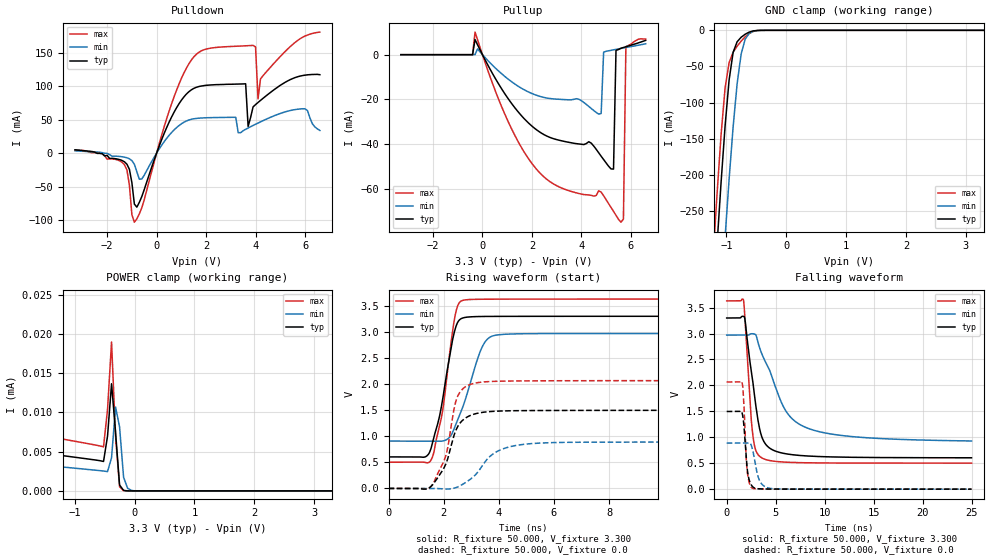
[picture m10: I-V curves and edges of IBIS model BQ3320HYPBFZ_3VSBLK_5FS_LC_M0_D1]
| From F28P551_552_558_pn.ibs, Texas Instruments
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|   Model BQ3320HYPBFZ_3VSBLK_5FS_LC_M0_D1
[Model] BQ3320HYPBFZ_3VSBLK_5FS_LC_M0_D1
Model_type I/O
Polarity   Non-Inverting
Enable   Active-Low
Vinl =  0.990V
Vinh =  2.310V
Vmeas =  1.650V
C_comp   3.470pF   3.136pF   3.588pF
[Model Spec]
Vinh   2.310V   2.079V   2.541V
Vinl   0.990V   0.891V   1.089V
Vmeas   1.650V   1.485V   1.815V
[Temperature Range]   25.000   0.155k   -40.000
[Voltage Range]   3.300V   2.970V   3.630V
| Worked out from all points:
|   slope of the pulldown table from 0 to 0.495 V, typ, clamps not added: 10.9 ohm
|   slope of the pullup table from 0 to 0.495 V, typ, clamps not added: 48.7 ohm
|   GND clamp passes 1 mA (typ) near -0.56 V on its own axis
|   rising waveform, R_fixture 50.000, V_fixture 3.300: 20-80 % time 559ps typ, 769ps min, 500ps max; typ from 0.605 V to 3.3 V
|   rising waveform, R_fixture 50.000, V_fixture 0.0: 20-80 % time 618ps typ, 974ps min, 527ps max; typ from 0 V to 1.5 V
|   falling waveform, R_fixture 50.000, V_fixture 3.300: 20-80 % time 1.21ns typ, 3.11ns min, 663ps max; typ from 3.3 V to 0.605 V
|   falling waveform, R_fixture 50.000, V_fixture 0.0: 20-80 % time 391ps typ, 623ps min, 307ps max; typ from 1.5 V to 0 V
[Pulldown]
|Voltage   I(typ)   I(min)   I(max)
-3.3V     4.876mA    3.346mA    4.743mA
-1.3V     -13.05mA   -6.062mA   -17.42mA
-900mV    -76.2mA    -16.7mA    -103.3mA
-600mV    -64.99mA   -38.74mA   -81.7mA
700mV     60.75mA    34.43mA    83.66mA
1.6V      98.27mA    51.81mA    147.5mA
3.6V      103.6mA    35.59mA    160.4mA
3.7V      39.88mA    37.53mA    160.6mA
4V        72.48mA    43.12mA    158.8mA
4.1V      75.66mA    44.92mA    80.91mA
6V        116.5mA    66.27mA    175mA
6.6V      117.2mA    33.86mA    180.9mA
[Pullup]
|Voltage   I(typ)   I(min)   I(max)
-3.3V     91.12nA    732.4nA    262.6pA
-300mV    6.771mA    40uA       10.12mA
2.1V      -32.9mA    -17.84mA   -50.16mA
4.7V      -43.94mA   -26.62mA   -60.94mA
4.8V      -45.49mA   -26.33mA   -61.57mA
4.9V      -46.98mA   1.13mA     -63.18mA
5.3V      -51.24mA   2.168mA    -70.17mA
5.4V      1.932mA    2.379mA    -71.96mA
5.6V      2.89mA     2.795mA    -75.03mA
5.7V      3.22mA     3.001mA    -73.63mA
5.8V      3.551mA    3.206mA    3.599mA
6.6V      6.407mA    4.882mA    7.034mA
[GND_clamp]
|Voltage   I(typ)   I(min)   I(max)
-3.3V     -3.505A    -3.628A    -3.476A
-1.223V   -386.4mA   -550.8mA   -315.4mA
-1.156V   -296.3mA   -460mA     -226.1mA
-1.089V   -210.5mA   -371.5mA   -144.6mA
-1.022V   -132.4mA   -286.5mA   -79.77mA
-955mV    -68.78mA   -206.3mA   -44.76mA
-888mV    -30.47mA   -133.9mA   -30.31mA
-821mV    -15.84mA   -73.99mA   -22.01mA
-754mV    -9.591mA   -32.92mA   -15.01mA
-687mV    -5.432mA   -12.28mA   -9.043mA
-620mV    -2.525mA   -4.288mA   -4.466mA
3.3V      0A         0A         0A
[POWER_clamp]
|Voltage   I(typ)   I(min)   I(max)
-3.3V     514.6uA    72.31mA    9.489uA
-3.266V   143.9uA    52.63mA    9.442uA
-3.132V   7.182uA    5.855mA    9.258uA
-2.931V   6.231uA    34.42uA    8.983uA
-2.864V   6.164uA    9.16uA     8.891uA
-2.73V    6.03uA     4.29uA     8.707uA
-519mV    3.757uA    2.535uA    5.612uA
-385mV    13.66uA    4.234uA    18.99uA
-318mV    7.479uA    10.7uA     6.925uA
-251mV    757.2nA    8.165uA    518.6nA
-184mV    65.2nA     1.742uA    33.01nA
3.3V      0A         0A         0A
[Ramp]
| variable   typ   min   max
dV/dt_r   0.899/0.618n   0.533/0.974n   1.240/0.527n
dV/dt_f   1.617/1.213n   1.225/3.112n   1.876/0.663n
R_load = 50.000
[Rising Waveform]
R_fixture= 50.000
V_fixture= 3.300
V_fixture_min= 2.970
V_fixture_max= 3.630
|time   V(typ)   V(min)   V(max)
0s        604.5mV    907.6mV    502.5mV
1.305ns   601.3mV    908.1mV    500.8mV
1.574ns   835.9mV    908.1mV    579.4mV
1.964ns   1.72V      908.9mV    1.501V
2.415ns   3.055V     1.195V     3.317V
2.544ns   3.214V     1.369V     3.543V
2.715ns   3.271V     1.594V     3.608V
3.389ns   3.296V     2.704V     3.627V
3.958ns   3.298V     2.943V     3.628V
25ns      3.3V       2.97V      3.63V
[Rising Waveform]
R_fixture= 50.000
V_fixture= 0.0
V_fixture_min= 0.0
V_fixture_max= 0.0
|time   V(typ)   V(min)   V(max)
0s        2.237uV    2.235uV    1.89uV
1.529ns   34.78mV    929.9uV    27.26mV
2.082ns   475.6mV    -12.54mV   637.8mV
2.373ns   1.017V     4.41mV     1.519V
2.506ns   1.186V     28.01mV    1.767V
2.778ns   1.345V     108.5mV    1.945V
3.233ns   1.442V     310mV      2.028V
3.997ns   1.483V     724.9mV    2.055V
5.517ns   1.494V     870.4mV    2.063V
25ns      1.498V     888.2mV    2.066V
[Falling Waveform]
R_fixture= 50.000
V_fixture= 3.300
V_fixture_min= 2.970
V_fixture_max= 3.630
|time   V(typ)   V(min)   V(max)
0s        3.3V       2.97V      3.63V
1.718ns   3.331V     2.97V      3.647V
1.872ns   3.269V     2.97V      3.262V
2.401ns   2.419V     2.99V      1.611V
2.634ns   2.116V     2.997V     1.101V
2.954ns   1.64V      2.98V      758mV
3.515ns   1.05V      2.644V     611.4mV
5.917ns   686.5mV    1.547V     521.6mV
7.997ns   642.6mV    1.197V     509.2mV
25ns      605.1mV    929.1mV    502.6mV
[Falling Waveform]
R_fixture= 50.000
V_fixture= 0.0
V_fixture_min= 0.0
V_fixture_max= 0.0
|time   V(typ)   V(min)   V(max)
0s        1.498V     888.2mV    2.066V
1.586ns   1.462V     888.1mV    2.05V
1.719ns   1.302V     888.1mV    1.791V
1.938ns   733.7mV    888mV      777.1mV
2.062ns   446.7mV    888mV      413.2mV
2.309ns   170.8mV    894.7mV    119.8mV
2.639ns   49.82mV    765.2mV    17.82mV
3.329ns   6.822mV    177.2mV    4.528mV
4.385ns   2.435mV    17.43mV    2.169mV
25ns      13.26uV    52.33uV    22.28uV
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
